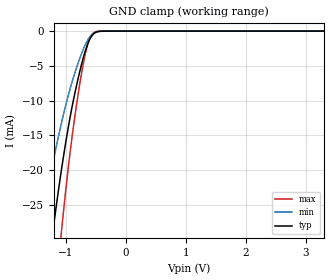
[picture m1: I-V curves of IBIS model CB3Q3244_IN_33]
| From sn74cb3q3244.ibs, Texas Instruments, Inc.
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[Model]   CB3Q3244_IN_33
Model_type  Input
Vinl=0.8
Vinh=2.0
| variable   typ   min   max
C_comp   2.07pF   1.67pF   3.12pF
[Temperature Range]   40   100   -40
| Ambient temperature   25   85   -40
[Voltage range]   3.3   3   3.6
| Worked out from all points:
|   GND clamp passes 1 mA (typ) near -0.59 V on its own axis
[GND Clamp]
| CB3Q3244_IN_33
|   Voltage   I(typ)   I(min)   I(max)
-5.5V     -449.5mA   -341.7mA   -565mA
-1.43V    -44.06mA   -29.15mA   -63.9mA
-1.405V   -42.18mA   -27.88mA   -61.24mA
-1.22V    -29.1mA    -19.19mA   -42.44mA
-1.08V    -20.38mA   -13.49mA   -29.49mA
-1.06V    -19.23mA   -12.75mA   -27.76mA
-975mV    -14.66mA   -9.782mA   -20.85mA
-900mV    -11.09mA   -7.448mA   -15.49mA
-765mV    -5.728mA   -3.865mA   -7.454mA
-640mV    -1.968mA   -1.351mA   -2.059mA
-535mV    -381.1uA   -297.7uA   -232.2uA
3.3V      204.1pA    546.3pA    112.7pA
